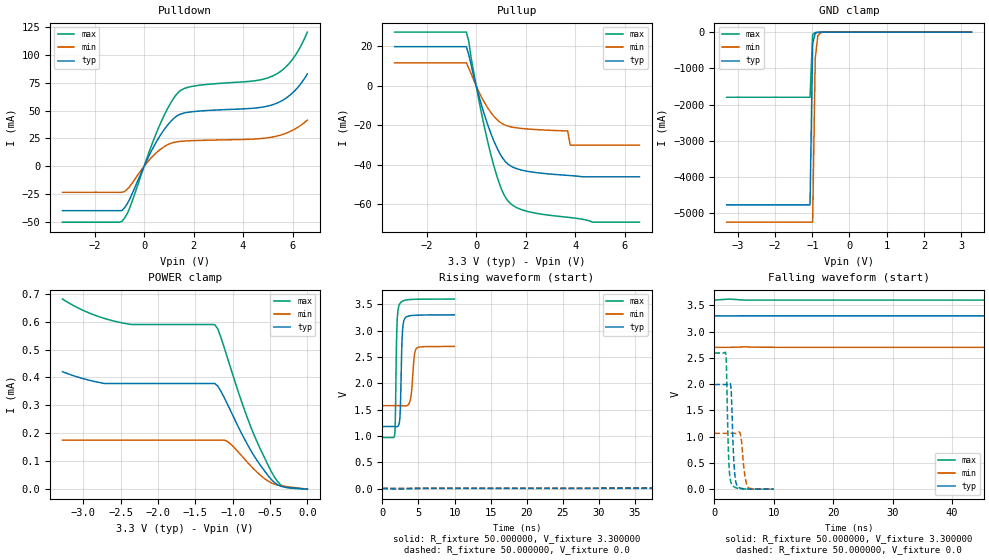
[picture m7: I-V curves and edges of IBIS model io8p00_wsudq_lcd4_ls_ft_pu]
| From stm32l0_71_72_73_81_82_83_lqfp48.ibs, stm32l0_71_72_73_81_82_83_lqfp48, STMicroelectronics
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|   Model io8p00_wsudq_lcd4_ls_ft_pu
[Model]  io8p00_wsudq_lcd4_ls_ft_pu
Model_type I/O
Polarity   Non-Inverting
Enable   Active-Low
Vinl =   0.990000V
Vinh =   2.310000V
Vmeas =  1.650000V
Cref =   50.000000pF
Rref =   100.000000M
Vref =   0.0V
C_comp   3.263700pF   3.224700pF   3.309000pF
[Temperature Range]   25.000000   0.125000k   -40.000000
[Pullup Reference]   3.300000V   2.700000V   3.600000V
[Pulldown Reference]   0.0V   0.0V   0.0V
[POWER Clamp Reference]   3.300000V   2.700000V   3.600000V
[GND Clamp Reference]   0.0V   0.0V   0.0V
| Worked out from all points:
|   slope of the pulldown table from 0 to 0.495 V, typ, clamps not added: 22.6 ohm
|   slope of the pullup table from 0 to 0.495 V, typ, clamps not added: 23.9 ohm
|   GND clamp passes 1 mA (typ) near -0.64 V on its own axis
|   rising waveform, R_fixture 50.000000, V_fixture 3.300000: 20-80 % time 236ps typ, 378ps min, 200ps max; typ from 1.18 V to 3.3 V
|   rising waveform, R_fixture 50.000000, V_fixture 0.0: 20-80 % time 204ns typ, 424ns min, 99.3ns max; typ from 0.001 V to 1.99 V
|   falling waveform, R_fixture 50.000000, V_fixture 3.300000: 20-80 % time 191ns typ, 380ns min, 105ns max; typ from 3.3 V to 1.18 V
|   falling waveform, R_fixture 50.000000, V_fixture 0.0: 20-80 % time 419ps typ, 581ps min, 343ps max; typ from 1.99 V to 0.001 V
[Pulldown]
|Voltage   I(typ)   I(min)   I(max)
-3.3V     -39.83mA   -23.37mA   -50.2mA
-900mV    -39.83mA   -23.37mA   -49.52mA
-600mV    -30.28mA   -18.59mA   -38.45mA
100mV     4.867mA    2.821mA    6.48mA
600mV     25.85mA    14.17mA    35.39mA
1V        38.33mA    19.81mA    53.88mA
1.4V      46.1mA     22.18mA    66.72mA
2V        49.07mA    23.02mA    71.93mA
4.4V      52.05mA    24.38mA    76.53mA
5.2V      55.25mA    26.3mA     81.02mA
6V        65.78mA    32.24mA    95.96mA
6.6V      82.83mA    41.41mA    120.4mA
[Pullup]
|Voltage   I(typ)   I(min)   I(max)
-3.3V     19.9mA     11.73mA    27.27mA
-400mV    19.9mA     11.73mA    27.27mA
-300mV    15.74mA    8.978mA    22.52mA
200mV     -9.115mA   -5.294mA   -12.98mA
600mV     -24.29mA   -13.56mA   -35.12mA
1V        -35.2mA    -18.69mA   -51.63mA
1.4V      -40.6mA    -20.72mA   -59.71mA
2.1V      -43.28mA   -21.83mA   -63.62mA
3.7V      -45.29mA   -22.8mA    -66.51mA
3.8V      -45.39mA   -30mA      -66.64mA
4.7V      -46.01mA   -30mA      -69mA
6.6V      -46.01mA   -30mA      -69mA
[GND_clamp]
|Voltage   I(typ)   I(min)   I(max)
-3.3V     -4.767A    -5.245A    -1.798A
-1.06V    -4.767A    -5.245A    -1.798A
-990mV    -327.3mA   -5.245A    -68.38mA
-920mV    -29.22mA   -722.7mA   -11.24mA
-850mV    -6.771mA   -104.4mA   -6.721mA
-780mV    -3.56mA    -17.38mA   -4.326mA
-500mV    -59.41uA   -172uA     -34.91uA
3.28V     0A         0A         0A
[POWER_clamp]
|Voltage   I(typ)   I(min)   I(max)
-3.28V    420.5uA    175.8uA    680.7uA
-2.72V    378.4uA    175.8uA    611.5uA
-2.4V     378.3uA    175.8uA    591.3uA
-1.24V    378.3uA    175.8uA    588.9uA
-1.2V     368.9uA    175.8uA    573.6uA
-1.08V    309.6uA    172.2uA    478.3uA
-920mV    220.5uA    131.5uA    344.5uA
-760mV    139.7uA    83.77uA    224.7uA
-480mV    33.95uA    22.2uA     61.82uA
-400mV    15.86uA    14.75uA    27.74uA
-320mV    8.148uA    10.83uA    9.341uA
0V        0A         0A         0A
[Ramp]
| variable   typ   min   max
dV/dt_r  1.19492/0.20377u   0.61277/0.42619u   1.55547/99.19330n
dV/dt_f  1.27230/0.19092u   0.63588/0.38002u   1.57816/0.10494u
R_load = 50.000000
[Rising Waveform]
R_fixture= 50.000000
V_fixture= 3.300000
V_fixture_min= 2.700000
V_fixture_max= 3.600000
|time   V(typ)   V(min)   V(max)
0s        1.178V     1.575V     969.7mV
1.702ns   1.177V     1.575V     1.017V
1.802ns   1.176V     1.575V     1.359V
2.022ns   1.174V     1.575V     3.086V
2.382ns   1.278V     1.575V     3.504V
2.743ns   2.869V     1.574V     3.556V
3.063ns   3.219V     1.57V      3.576V
3.884ns   3.284V     1.687V     3.591V
4.725ns   3.293V     2.662V     3.596V
9.97ns    3.3V       2.7V       3.6V
[Rising Waveform]
R_fixture= 50.000000
V_fixture= 0.0
V_fixture_min= 0.0
V_fixture_max= 0.0
|time   V(typ)   V(min)   V(max)
0s        1.061mV    1.817mV    656.1uV
47.55ns   4.081mV    4.548mV    67.91mV
100.1ns   82.06mV    4.582mV    927.8mV
165.2ns   466.2mV    11.11mV    1.944V
205.2ns   756.9mV    21.09mV    2.298V
252.8ns   1.082V     58.27mV    2.483V
367.9ns   1.624V     213.8mV    2.577V
498ns     1.878V     441.1mV    2.591V
790.8ns   1.984V     850.6mV    2.593V
1.246us   1.993V     1.064V     2.593V
[Falling Waveform]
R_fixture= 50.000000
V_fixture= 3.300000
V_fixture_min= 2.700000
V_fixture_max= 3.600000
|time   V(typ)   V(min)   V(max)
0s        3.3V       2.7V       3.6V
82.58ns   3.3V       2.7V       3.49V
150.2ns   3.19V      2.7V       2.487V
212.7ns   2.837V     2.697V     1.576V
250.2ns   2.577V     2.686V     1.219V
290.3ns   2.289V     2.661V     1.073V
395.4ns   1.614V     2.545V     996.7mV
498ns     1.332V     2.373V     979.2mV
830.8ns   1.196V     1.786V     970.3mV
1.246us   1.178V     1.575V     969.7mV
[Falling Waveform]
R_fixture= 50.000000
V_fixture= 0.0
V_fixture_min= 0.0
V_fixture_max= 0.0
|time   V(typ)   V(min)   V(max)
0s        1.993V     1.064V     2.593V
1.922ns   1.993V     1.064V     2.565V
2.402ns   1.998V     1.064V     555.6mV
2.863ns   1.77V      1.064V     103.5mV
3.303ns   461.2mV    1.064V     46.84mV
3.784ns   75.46mV    1.069V     21.32mV
4.384ns   20.92mV    1.04V      8.444mV
5.045ns   8.508mV    317mV      4.737mV
5.666ns   4.787mV    39.15mV    3.413mV
9.97ns    1.061mV    1.817mV    656.1uV
